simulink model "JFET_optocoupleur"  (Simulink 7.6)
settings: Solver=ode15s  StartTime=0.0  StopTime=10.0  RelTol=1e-3
libraries: fl_lib x5, elec_lib x5, nesl_utility x2

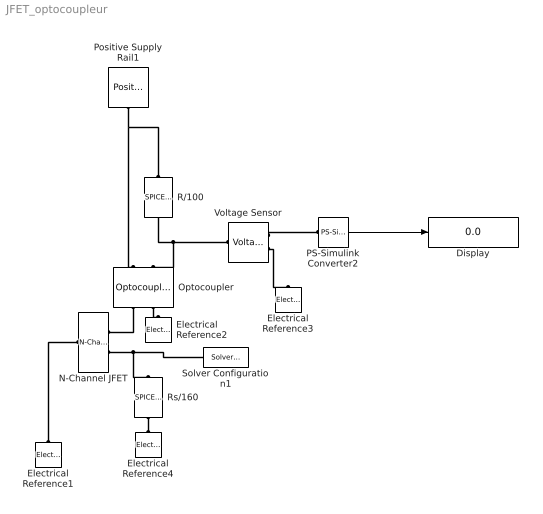
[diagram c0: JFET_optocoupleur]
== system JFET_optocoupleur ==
  Display : Display
  Electrical Reference{1..4} (4 alike) : fl_lib/Electrical/Electrical Elements/Electrical Reference  DialogController=NetworkEngine.DynNeDlgSource  SystemSampleTime=-1  i_Log=off  LocalVarNames=|i  LocalVarDescs=|i  LocalVarLogging=[]
  N-Channel JFET : elec_lib/Semiconductor Devices/N-Channel JFET  DialogController=NetworkEngine.DynNeDlgSource  SystemSampleTime=-1  parameterization=1  Igss=-1 nA  Idss=17 mA  Idss_v="[  0 15 ] V"  ssig="[  3e+03 10 ] uS"  ssig_v="[  0 15 ] V"  Beta=1e-04 A/V^2  IS=1e-14 A  Tmeas=25 C  Vt0=-2 V  Lchannel=0 1/V  RS=0.1 Ohm  RD=0.1 Ohm  C_param=1  C_GS=3 pF  C_GD=1.5 pF  C_iss=4.5 pF  C_rss=1.5 pF  LocalVarLogging=[]
  Optocoupler : elec_lib/Semiconductor Devices/Optocoupler  DialogController=NetworkEngine.DynNeDlgSource  SystemSampleTime=-1  CTR=0.2  prmExp=1  I12="[  0.001 0.015 ] A"  V12="[  0.9 1.05 ] V"  RS=0.1 Ohm  IS=1e-10 A  Tmeas=25 C  ec=2  C_param=1  CJ0=5 pF  VJ=1 V  Mgrad=0.5  Vvec="[  0.1 10 100 ] V"  Cvec="[  3.5 1 0.4 ] pF"  FC=0.5  LocalVarLogging=[]
  PS-Simulink Converter2 : nesl_utility/PS-Simulink Converter  DialogController=NetworkEngine.DynNeUtilDlgSource  SystemSampleTime=-1  PhysicalDomain=network_engine_domain  LeftPortType=input  RightPortType=output  SubClassName=ps_output  Unit=1  AffineConversion=off
  Positive Supply Rail1 : elec_lib/Sources/Positive Supply Rail  DialogController=NetworkEngine.DynNeDlgSource  SystemSampleTime=-1  v0=15 V  current_Log=off  voltage_Log=off  power_Log=off  LocalVarNames=|current|voltage|power  LocalVarDescs=|Current (A)|Voltage (V)|Power (W)  LocalVarLogging=[0 0 0]
  R/100 : elec_lib/Additional Components/SPICE-Compatible Components/Passive Devices/SPICE Resistor  DialogController=NetworkEngine.DynNeDlgSource  SystemSampleTime=-1  SCALE=1  R_param=1  R=100 Ohm  RSH=0 Ohm  LENGTH=1e-06 m  WIDTH=1e-06 m  NARROW=0 m  T_param=1  TC1=0 1/K  TC2=0 1/K^2  TOFFSET=0 K  TFIXED=300.15 K  TMEAS=300.15 K  LocalVarLogging=[]
  Rs/160 : elec_lib/Additional Components/SPICE-Compatible Components/Passive Devices/SPICE Resistor  DialogController=NetworkEngine.DynNeDlgSource  SystemSampleTime=-1  SCALE=1  R_param=1  R=160 Ohm  RSH=0 Ohm  LENGTH=1e-06 m  WIDTH=1e-06 m  NARROW=0 m  T_param=1  TC1=0 1/K  TC2=0 1/K^2  TOFFSET=0 K  TFIXED=300.15 K  TMEAS=300.15 K  LocalVarLogging=[]
  Solver Configuration1 : nesl_utility/Solver Configuration  DialogController=NetworkEngine.DynNeUtilDlgSource  SystemSampleTime=-1  PhysicalDomain=network_engine_domain  LeftPortType=input  RightPortType=generic  SubClassName=solver  Accelerate=off  Profile=off  ResidualTolerance=1e-9  MaxNonlinIter=12  MaxModeIter=2  DoFixedCost=off  UseLocalSampling=off  DoDC=off  LinearAlgebra=Sparse  LocalSolverSampleTime=.001  LocalSolverChoice=NE_BACKWARD_EULER_ADVANCER  UseLocalSolver=off
  Voltage Sensor : fl_lib/Electrical/Electrical Sensors/Voltage Sensor  DialogController=NetworkEngine.DynNeDlgSource  SystemSampleTime=-1  i1_Log=off  v1_Log=off  LocalVarNames=|i1|v1  LocalVarDescs=|i1|v1  LocalVarLogging=[0 0]
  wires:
  PS-Simulink Converter2/1 -> Display/1
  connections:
  Rs/160/RConn1 -- Electrical Reference4/LConn1
  N-Channel JFET/RConn2 -- Rs/160/LConn1 -- Solver Configuration1/RConn1
  Positive Supply Rail1/RConn1 -- Optocoupler/LConn1 -- R/100/LConn1
  Optocoupler/RConn1 -- N-Channel JFET/RConn1
  Electrical Reference1/LConn1 -- N-Channel JFET/LConn1
  Voltage Sensor/RConn2 -- Electrical Reference3/LConn1
  Voltage Sensor/RConn1 -- PS-Simulink Converter2/LConn1
  Optocoupler/RConn2 -- Electrical Reference2/LConn1
  Voltage Sensor/LConn1 -- Optocoupler/LConn2 -- R/100/RConn1
